FUNCTION_BLOCK FB 10
TITLE = FactoryLink H1 Encode
//KNOW_HOW_PROTECT
AUTHOR : DLink
FAMILY : S7_H1
NAME   : ENCODE
VERSION: 1.0

VAR_INPUT
  S5          : BOOL;                  // Trigger to start a WRITE operation
END_VAR

VAR
  Recv_Buf    : STRUCT                 // Receive buffer for a partners "Write" Reply
   Dest       : BYTE;                  // Destination
   Dtype      : BYTE;                  // Destination type
   DBno       : WORD;                  // DB number
   Address    : WORD;                  // Address (0 - 255)
   Bit        : BYTE;                  // Bit number
   Change     : BYTE;                  // Change marker
   V_low      : WORD;                  // Value low part
   V_high     : WORD;                  // Value high part
   Reserved   : DWORD;
  END_STRUCT;
END_VAR

VAR_TEMP
  Dest_Ptr    : ANY;                   // Pointer to the internal data buf with user data
  Adr         : DWORD;
  I_double    : DWORD;
  I_bit       : BOOL;
  I_byte      : BYTE;
  EN_STATUS   : BOOL;                  // Used only for EN, ENO operation
  Int_Var     : INT;                   // Temporary integer value
  Offset      : INT;
END_VAR


BEGIN
NETWORK
TITLE =

      SET   ;
      SAVE  ;
      =     #EN_STATUS;                // Save if any uses the EN, ENO status
      SET   ;                          // Make sure all info bits are zero
//
// Check if there is something to do
//
      L     #Recv_Buf.Change;
      L     0;
      ==I   ;
      JC    RDY;
      T     #Recv_Buf.Change;
//
// Evaluate encode write
//

      L     #Recv_Buf.Address;
      T     #Offset;
//
// Evaluate destination type
//
      L     77;                        // Flag byte destination
      L     #Recv_Buf.Dest;
      <>I   ;
      JC    D_DB;
      L     DW#16#8300_0000;           // Initialise address register
      T     #Adr;
      JU    CONT;
D_DB: L     68;                        // DB destination
      <>I   ;
      JC    D_QB;
      L     #Recv_Buf.DBno;
      T     #Int_Var;
      OPN   DB[#Int_Var];              // DB is now open
      L     DW#16#8400_0000;           // Initialise address register
      T     #Adr;
      AN    #S5;
      JC    CONT;
      L     #Offset;
      SLW   1;
      T     #Offset;
      L     82;                        // Data byte right type
      L     #Recv_Buf.Dtype;
      <>I   ;
      JC    LEFT;
      L     #Offset;
      L     +1;
      +I    ;
      T     #Offset;
      L     #Recv_Buf.V_low;
      SLW   8;
      T     #Recv_Buf.V_low;
      L     66;                        // Data byte changed to type byte
      T     #Recv_Buf.Dtype;
      JU    CONT;
LEFT: L     76;                        // Data type byte left
      <>I   ;
      JC    BIT;                       // Evaluate if type is bit
      L     66;                        // Data byte changed to type byte
      T     #Recv_Buf.Dtype;
      JU    CONT;
BIT:  L     70;                        // Data byte right type
      L     #Recv_Buf.Dtype;
      <>I   ;
      JC    CONT;                      // No specials for S5
      L     #Recv_Buf.Bit;
      L     8;                         // Check bit number
      <I    ;
      JC    ADD;
      -I    ;
      T     #Recv_Buf.Bit;             // Set bit number within byte
      JU    CONT;
ADD:  L     #Offset;
      L     +1;
      +I    ;
      T     #Offset;
      JU    CONT;
D_QB: L     65;                        // Ouput destination
      L     #Recv_Buf.Dest;
      <>I   ;
      JC    D_IB;
      L     DW#16#8200_0000;           // Initialise address register
      T     #Adr;
      JU    CONT;
D_IB: L     69;                        // Input destination
      <>I   ;
      JC    ERR;
      L     DW#16#8100_0000;           // Initialise address register
      T     #Adr;
      JU    CONT;
ERR:  NOP   0;
      JU    RDY;
CONT: L     #Offset;                   // Add address
      SLW   3;
      T     LW    12;
      L     #Adr;
      LAR1  ;
//
// Evaluate destination type
//
      L     70;                        // Flag type
      L     #Recv_Buf.Dtype;
      <>I   ;
      JC    T_B;
      L     7;
      L     #Recv_Buf.Bit;
      <I    ;
      JC    ERR;
      L     #Adr;
      +D    ;
      T     #Adr;
      LAR1  ;
      L     #Recv_Buf.V_low;
      L     0;
      <>I   ;
      =     [AR1,P#0.0];
      JU    RDY;
T_B:  L     66;                        // Byte type
      <>I   ;
      JC    T_W;
      L     #Recv_Buf.V_low;
      SRW   8;
      T     B[AR1,P#0.0];
      JU    RDY;
T_W:  L     87;                        // Word type
      L     #Recv_Buf.Dtype;
      <>I   ;
      JC    T_D;
      L     #Recv_Buf.V_low;
      T     W[AR1,P#0.0];
      JU    RDY;
T_D:  L     68;                        // Double type
      <>I   ;
      JC    RDY;
      L     #Recv_Buf.V_low;
      T     LW    14;
      L     #Recv_Buf.V_high;
      T     LW    16;
      L     #I_double;
      T     D[AR1,P#0.0];
RDY:  CLR   ;                          // restore the EN status to ENO
      A     #EN_STATUS;
      SAVE  ;
END_FUNCTION_BLOCK
